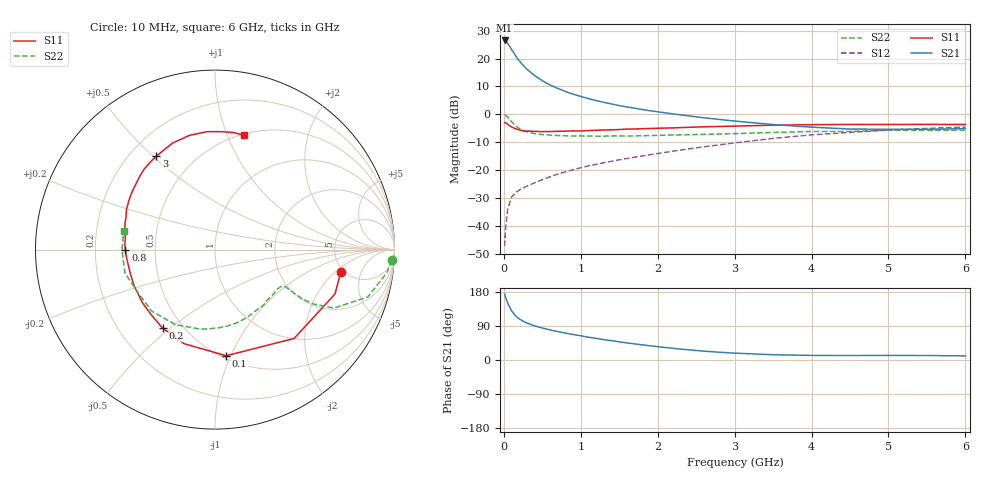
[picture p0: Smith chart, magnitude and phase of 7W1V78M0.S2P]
! Infineon Technologies  Discrete & RF Semiconductors
! BFS17W
! Si NPN RF Bipolar Junction Transistor in SOT323
! VCE = 1.75 V  IC = 8 mA
! Common Emitter S-Parameters:  August  1999
# GHz  S  MA  R  50
!  f  S11  S21  S12  S22
! GHz  MAG  ANG  MAG  ANG  MAG  ANG  MAG  ANG
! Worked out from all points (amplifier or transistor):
!   36 points, 10 MHz to 6 GHz, reference 50 ohm
!   highest |S21| = 26.5 dB at 10 MHz (marker M1)
!   |S21| within 3 dB of that: start of sweep to 95.35 MHz
!   unconditionally stable (mu >= 1): 411.7 MHz to 3.326 GHz; 3.713 GHz to end of sweep
!   at 250 MHz: K = 0.76, MSG = 22.1 dB, |S12| = -26.5 dB
!   at 1.4 GHz: K = 1.26, MAG = 7.2 dB, |S12| = -16.9 dB
!   at 6 GHz: K = 1.10, MAG = -2.2 dB, |S12| = -4.6 dB
!   S11 on the Smith chart (normalised r, x): 10 MHz: 4.67, -2.39; 100 MHz: 0.53, -0.96; 200 MHz: 0.39, -0.47; 800 MHz: 0.33, +0.00; 3 GHz: 0.31, +0.51; 6 GHz: 0.51, +1.15
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0.01  0.7117 -10.2  21.19 174.1  0.0043 83.7  0.9856 -3.4
0.02  0.713 -20.3  20.86 167.4  0.0083 82.4  0.9669 -7.6
0.05  0.6629 -48.3  18.89 150.2  0.0199 68.9  0.8914 -17.2
0.1  0.5947 -84.0  14.65 130.1  0.0327 57.1  0.738 -26.2
0.15  0.5517 -108.2  11.42 117.0  0.0388 50.9  0.624 -29.0
0.2  0.5261 -123.7  9.188 108.6  0.0436 50.3  0.5563 -29.4
0.25  0.507 -135.2  7.599 102.4  0.0473 49.0  0.5112 -28.9
0.3  0.5012 -143.6  6.465 97.6  0.0514 50.4  0.4837 -28.5
0.4  0.4937 -156.0  4.963 90.1  0.0591 53.0  0.4499 -27.9
0.5  0.4903 -164.3  4.023 84.4  0.0671 55.3  0.4339 -28.0
0.6  0.491 -170.3  3.372 79.5  0.0756 57.3  0.4236 -28.9
0.7  0.4956 -175.4  2.921 75.1  0.0845 58.7  0.417 -30.4
0.8  0.4991 180.0  2.577 71.0  0.0928 59.9  0.4121 -32.4
1.1  0.5117 169.1  1.914 60.2  0.1185 61.7  0.4077 -39.3
1.3  0.5234 163.0  1.642 53.8  0.1354 62.3  0.4055 -44.9
1.6  0.543 155.1  1.357 45.1  0.161 62.9  0.408 -53.8
2.2  0.5714 140.8  1.018 30.8  0.2182 62.8  0.4256 -73.4
3  0.6144 122.2  0.758 18.1  0.3076 59.2  0.4505 -100.4
3.5  0.6387 111.9  0.656 13.9  0.3698 54.8  0.4728 -117.8
4.5  0.6587 93.9  0.544 11.9  0.4732 42.5  0.4922 -151.8
5.5  0.6604 80.9  0.539 11.9  0.5583 30.7  0.5182 -179.4
6  0.6573 75.9  0.554 10.8  0.5921 25.0  0.5192 168.4
